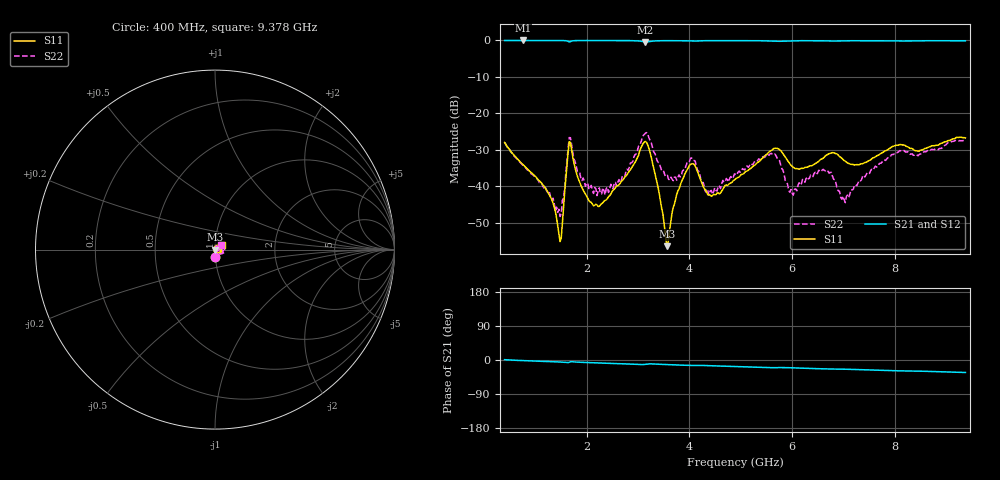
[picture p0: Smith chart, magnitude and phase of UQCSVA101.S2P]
!  Part Number  UQCSVA101  Mounting Orientation: Horizontal
!  Description: Ultra Low ESR Microwave capacitors
!  Application: Coupling, Bypass, Tuning, DC Block
!  Filters, Matching
# GHZ S DB R 50
! Freq  |S11|  S11 Ph  |S21|  S21 Ph  |S12|  S12 Ph  |S22|  S22 Ph
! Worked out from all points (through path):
!   400 points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, 400 MHz to 9.378 GHz, reference 50 ohm
!   highest |S21| = -0.01 dB at 760 MHz (marker M1); lowest = -0.4 dB at 3.145 GHz (marker M2)
!   group delay of S21, straight-line fit = 9.92 ps
!   lowest |S11| = -56.4 dB at 3.573 GHz (marker M3), VSWR 1.00, Z = 50.2 + j0.022 ohm
!   |S11| at or under -10 dB: start of sweep to end of sweep
!   |S22| runs from -48.2 to -25.3 dB; largest |S21 - S12| = 0.0054
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0.4  -27.98 -87.2  -0.02 0.8  0.00 0.8  -27.94 -87.0
0.76  -34.04 -89.3  -0.01 -1.6  -0.01 -1.6  -34.36 -88.5
1.323  -43.67 -109.5  -0.01 -4.4  -0.01 -4.5  -43.69 -72.4
1.48  -55.12 179.7  -0.02 -5.3  0.00 -5.3  -48.24 -32.0
1.66  -27.74 -2.4  -0.41 -6.0  -0.39 -6.0  -26.61 -9.2
1.908  -40.39 -116.0  -0.03 -6.2  -0.01 -6.3  -38.39 -67.5
2.133  -45.32 -160.0  -0.02 -7.3  -0.01 -7.4  -41.95 -45.2
2.425  -42.82 136.8  -0.03 -8.6  -0.01 -8.7  -41.67 -15.2
3.145  -27.69 5.3  -0.41 -11.4  -0.39 -11.5  -25.40 -1.3
3.393  -40.46 -64.5  -0.10 -11.1  -0.08 -11.2  -33.40 -39.3
3.573  -56.38 8.3  -0.06 -12.2  -0.05 -12.3  -36.97 -22.6
3.753  -42.22 62.9  -0.07 -13.1  -0.05 -13.2  -38.28 4.8
4.023  -33.93 23.9  -0.17 -14.2  -0.16 -14.3  -32.27 10.7
4.383  -42.27 0.2  -0.06 -15.0  -0.05 -15.1  -42.44 14.0
4.9  -37.97 35.0  -0.05 -17.3  -0.04 -17.4  -36.72 57.8
5.665  -29.56 8.8  -0.22 -20.2  -0.22 -20.4  -31.12 31.5
6.025  -34.75 -10.1  -0.11 -20.7  -0.10 -20.9  -42.39 54.4
6.408  -34.16 15.0  -0.08 -22.5  -0.08 -22.7  -37.31 73.9
6.768  -30.85 10.3  -0.16 -23.8  -0.16 -24.0  -36.20 40.3
7.038  -33.09 0.0  -0.12 -24.3  -0.12 -24.5  -44.44 67.4
7.893  -29.65 36.1  -0.10 -27.9  -0.11 -28.2  -32.16 42.0
9.378  -26.72 32.9  -0.10 -32.9  -0.12 -33.1  -27.51 36.2
